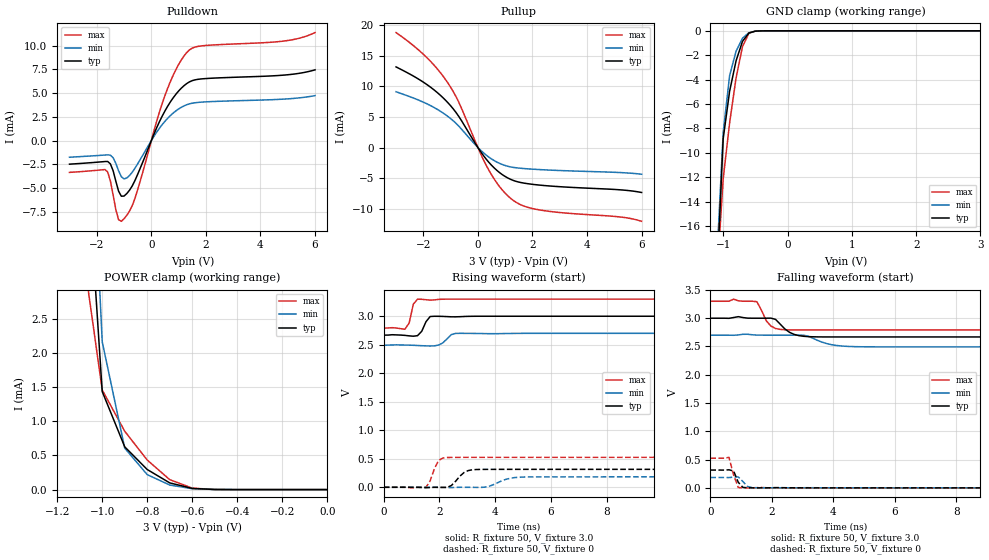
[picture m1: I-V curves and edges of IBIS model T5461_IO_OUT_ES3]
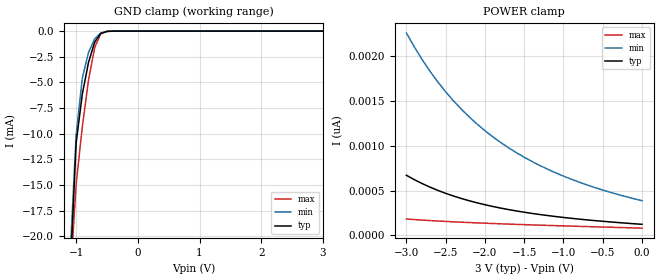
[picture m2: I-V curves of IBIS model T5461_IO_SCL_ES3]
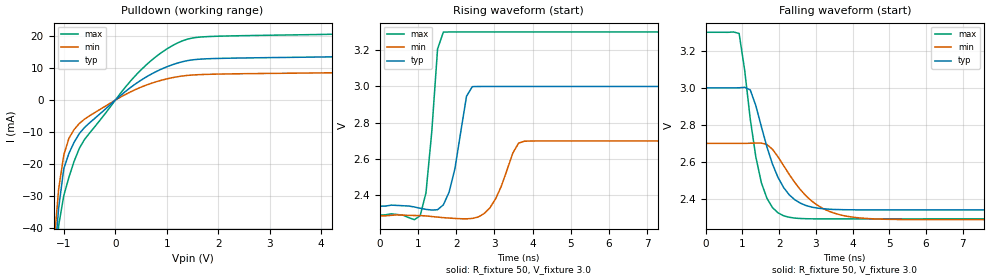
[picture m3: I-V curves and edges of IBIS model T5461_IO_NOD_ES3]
[IBIS Ver]   3.2
[Comment Char]   |_char
[File name]   rx8130ce_3v.ibs
[File Rev]   1.0
[Date]   2019/10/29 15:22:26
[Source]
[Notes]
[Disclaimer]
This information is for modeling purposes only, and is not guaranteed.
Property of SEIKO EPSON Corp.,
unauthorized reproduction and/or distribution is strictly prohibited.
[Copyright]
Copyright 2019, SEIKO EPSON Corp.
[Component]   T5461W0A0
Si_location Pin
Timing_location Pin
[Manufacturer]   SEIKO EPSON Corp.
| RX8130CE
[Package]
R_pkg   0.0m   0.0m   0.0m
L_pkg   0.0n   0.0n   0.0n
C_pkg   0.0p   0.0p   0.0p
[Pin] signal_name   model_name
1   VIO   POWER
2   SCL   T5461_IO_SCL_ES3
3   SDA   T5461_IO_DIO_SMT_ES3
4   FOUT   T5461_IO_OUT_ES3
5   /RST   T5461_IO_NOD_ES3
6   /IRQ   T5461_IO_NOD_ES3
7   GND   POWER
8   VDD   POWER
9   VOUT   POWER
10   VBAT   POWER
| Models and submodels in the file (4): T5461_IO_OUT_ES3 (3-state), T5461_IO_SCL_ES3 (Input), T5461_IO_NOD_ES3 (Open_drain), T5461_IO_DIO_SMT_ES3 (I/O_open_drain)
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[Model]   T5461_IO_OUT_ES3
Model_type 3-state
Enable Active-High
Polarity Non-Inverting
Vmeas=1.50
C_comp   2.5p   2.0p   3.0p
[Temperature Range] 25   85   -40
[Voltage Range]   3.0   2.7   3.3
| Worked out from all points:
|   slope of the pulldown table from 0 to 0.45 V, typ, clamps not added: 157 ohm
|   slope of the pullup table from 0 to 0.45 V, typ, clamps not added: 170 ohm
|   GND clamp passes 1 mA (typ) near -0.71 V on its own axis
|   POWER clamp passes 1 mA (typ) near -0.95 V on its own axis
|   falling waveform, R_fixture 50, V_fixture 3.0: 20-80 % time 437ps typ, 644ps min, 312ps max; typ from 3 V to 2.67 V
|   falling waveform, R_fixture 50, V_fixture 0: 20-80 % time 175ps typ, 196ps min, 177ps max; typ from 0.315 V to 0 V
|   rising waveform, R_fixture 50, V_fixture 3.0: 20-80 % time 204ps typ, 261ps min, 138ps max; typ from 2.67 V to 3 V
|   rising waveform, R_fixture 50, V_fixture 0: 20-80 % time 372ps typ, 557ps min, 264ps max; typ from 0 V to 0.315 V
[Pullup]
-3V       13.15mA    9.1mA      18.76mA
-2V       10.67mA    7.402mA    15.22mA
-1.2V     7.774mA    5.394mA    11.17mA
-700mV    5.069mA    3.488mA    7.383mA
100mV     -670.8uA   -442.9uA   -1.015mA
400mV     -2.405mA   -1.562mA   -3.683mA
800mV     -4.114mA   -2.598mA   -6.416mA
1.3V      -5.375mA   -3.246mA   -8.638mA
1.7V      -5.817mA   -3.436mA   -9.577mA
2.3V      -6.149mA   -3.611mA   -10.21mA
5.2V      -6.899mA   -4.083mA   -11.33mA
6V        -7.339mA   -4.363mA   -12.04mA
[Pulldown]
-3V       -2.479mA   -1.747mA   -3.344mA
-1.6V     -2.194mA   -1.497mA   -3.304mA
-1.4V     -3.175mA   -1.806mA   -5.728mA
-1.2V     -5.321mA   -3.18mA    -8.323mA
-1.1V     -5.852mA   -3.796mA   -8.495mA
-900mV    -5.578mA   -3.932mA   -7.863mA
-600mV    -4.197mA   -2.907mA   -6.073mA
600mV     3.627mA    2.353mA    5.517mA
1.3V      6.014mA    3.781mA    9.282mA
1.8V      6.487mA    4.045mA    9.961mA
4.8V      6.886mA    4.362mA    10.47mA
6V        7.452mA    4.738mA    11.38mA
[GND Clamp]
-3V       -430mA     -359.3mA   -539.8mA
-1.1V     -20.64mA   -18.88mA   -20.39mA
-1V       -8.831mA   -8.329mA   -12.11mA
-900mV    -4.941mA   -3.657mA   -7.543mA
-800mV    -2.459mA   -1.675mA   -3.865mA
-700mV    -864uA     -604.2uA   -1.29mA
-600mV    -179.4uA   -151uA     -195.7uA
-500mV    -26.95uA   -29.51uA   -18.23uA
-400mV    -3.685uA   -4.954uA   -1.653uA
3V        88.91pA    20.06nA    44.45pA
[POWER Clamp]
-3V       324.7mA    274.7mA    407.4mA
-1.1V     6.482mA    9.074mA    3.807mA
-1V       1.434mA    2.163mA    1.457mA
-900mV    625.6uA    606.7uA    853.6uA
-800mV    293.7uA    218.9uA    432uA
-700mV    98.19uA    66.89uA    145.6uA
-600mV    17.36uA    13.33uA    21.68uA
-500mV    1.719uA    1.888uA    1.298uA
0V        88.91pA    301.9pA    52.79pA
[Falling Waveform]
R_fixture=50
V_fixture=3.0
V_fixture_min=2.7
V_fixture_max=3.3
0s        3V         2.7V       3.3V
1.515ns   3V         2.702V     3.292V
1.818ns   3V         2.7V       2.957V
1.97ns    3.001V     2.7V       2.862V
2.121ns   2.979V     2.7V       2.819V
2.424ns   2.811V     2.7V       2.796V
3.03ns    2.681V     2.699V     2.793V
3.939ns   2.669V     2.532V     2.793V
4.697ns   2.668V     2.497V     2.793V
15ns      2.668V     2.493V     2.793V
[Falling Waveform]
R_fixture=50
V_fixture=0
V_fixture_min=0
V_fixture_max=0
0s        314.7mV    183mV      525mV
454.5ps   313.6mV    182.4mV    523.9mV
606.1ps   319.2mV    181.5mV    540.1mV
757.6ps   298.7mV    190.7mV    227.4mV
909.1ps   98.15mV    193.1mV    5.762mV
1.061ns   8.292mV    110.5mV    366.7uV
1.212ns   925.4uV    24.36mV    -21.8uV
1.364ns   103.2uV    4.285mV    329.5uV
1.515ns   -16.13uV   1.324mV    4.103mV
15ns      0V         0V         0V
[Rising Waveform]
R_fixture=50
V_fixture=3.0
V_fixture_min=2.7
V_fixture_max=3.3
0s        2.668V     2.493V     2.793V
757.6ps   2.664V     2.495V     2.772V
909.1ps   2.656V     2.493V     2.877V
1.061ns   2.65V      2.49V      3.212V
1.212ns   2.659V     2.487V     3.299V
1.364ns   2.736V     2.483V     3.297V
1.667ns   2.995V     2.478V     3.283V
1.818ns   2.999V     2.48V      3.287V
2.576ns   2.99V      2.699V     3.3V
15ns      3V         2.7V       3.3V
[Rising Waveform]
R_fixture=50
V_fixture=0
V_fixture_min=0
V_fixture_max=0
0s        0V         0V         0V
1.515ns   -8.195mV   111.8uV    440.3uV
1.667ns   -4.303mV   98.36uV    115mV
1.818ns   -472.6uV   -134.8uV   326.9mV
1.97ns    -1.214mV   -804.1uV   468.6mV
2.273ns   -1.665mV   -4.03mV    521.9mV
2.879ns   257.7mV    -371uV     524.6mV
3.333ns   311.7mV    -2.063mV   524.9mV
5ns       314.7mV    179.3mV    525mV
15ns      314.7mV    183mV      525mV
[Ramp]
R_load=50
dV/dt_r   1.888E-1/3.592E-10   1.098E-1/5.448E-10   3.150E-1/2.380E-10
dV/dt_f   1.989E-1/4.212E-10   1.243E-1/6.375E-10   3.044E-1/2.762E-10
|[End   T5461_IO_OUT_ES3
[Model]   T5461_IO_SCL_ES3
Model_type Input
Enable Active-High
Polarity Non-Inverting
Vinh=2.64
Vinl=0.54
C_comp   2.5p   2.0p   3.0p
[Temperature Range] 25   85   -40
[Voltage Range]   3.0   2.7   3.3
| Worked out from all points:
|   GND clamp passes 1 mA (typ) near -0.69 V on its own axis
[GND Clamp]
-3V       -502.2mA   -418.5mA   -628.9mA
-1.1V     -24.07mA   -22.18mA   -24.54mA
-1V       -10.87mA   -10.09mA   -14.91mA
-900mV    -6.13mA    -4.561mA   -9.309mA
-800mV    -3.058mA   -2.097mA   -4.786mA
-700mV    -1.078mA   -757.4uA   -1.604mA
-600mV    -224.6uA   -189.6uA   -244.1uA
-500mV    -33.81uA   -37.1uA    -22.82uA
-400mV    -4.624uA   -6.222uA   -2.07uA
3V        124.1pA    455.9pA    73.37pA
[POWER Clamp]
-3V       672pA      2.262nA    183.3pA
-2.8V     579.6pA    1.965nA    171.4pA
-2.7V     539.7pA    1.834nA    166pA
-2.5V     470.3pA    1.605nA    156.4pA
-2.4V     440.2pA    1.503nA    152pA
-2.2V     387.4pA    1.324nA    143.9pA
-2V       343.1pA    1.17nA     136.5pA
-1.8V     305.5pA    1.039nA    129.8pA
-1.4V     245.9pA    825.7pA    117.6pA
-1V       200.8pA    662.6pA    106.6pA
-500mV    157.9pA    507.1pA    93.84pA
0V        124.1pA    388pA      81.19pA
[Model]   T5461_IO_NOD_ES3
Model_type Open_drain
Enable Active-High
Polarity Non-Inverting
Vmeas=1.50
Vref=3.3
Rref=5000
C_comp   2.5p   2.0p   3.0p
[Temperature Range] 25   85   -40
[Voltage Range]   3.0   2.7   3.3
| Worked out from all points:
|   slope of the pulldown table from 0 to 0.45 V, typ, clamps not added: 78.7 ohm
|   falling waveform, R_fixture 50, V_fixture 3.0: 20-80 % time 679ps typ, 1.01ns min, 450ps max; typ from 3 V to 2.34 V
|   rising waveform, R_fixture 50, V_fixture 3.0: 20-80 % time 332ps typ, 458ps min, 231ps max; typ from 2.34 V to 3 V
[Pulldown]
-3V       -460.3mA   -383.6mA   -577.8mA
-1.2V     -53.34mA   -46.96mA   -63.7mA
-1.1V     -33.78mA   -27.79mA   -39.25mA
-1V       -21.42mA   -17.13mA   -29.89mA
-900mV    -16.66mA   -11.93mA   -24.12mA
-700mV    -10.51mA   -7.336mA   -15.14mA
-600mV    -8.596mA   -5.984mA   -12.36mA
500mV     6.256mA    4.072mA    9.496mA
900mV     9.765mA    6.259mA    14.95mA
1.3V      12.03mA    7.562mA    18.56mA
1.8V      12.97mA    8.09mA     19.92mA
6V        14.9mA     9.477mA    22.76mA
[Falling Waveform]
R_fixture=50
V_fixture=3.0
V_fixture_min=2.7
V_fixture_max=3.3
0s        3V         2.7V       3.3V
909.1ps   3V         2.7V       3.293V
1.061ns   3.003V     2.7V       3.094V
1.212ns   2.989V     2.701V     2.832V
1.515ns   2.79V      2.701V     2.487V
1.818ns   2.588V     2.668V     2.353V
2.121ns   2.462V     2.58V      2.309V
3.03ns    2.351V     2.368V     2.292V
4.091ns   2.341V     2.3V       2.292V
15ns      2.341V     2.288V     2.292V
[Rising Waveform]
R_fixture=50
V_fixture=3.0
V_fixture_min=2.7
V_fixture_max=3.3
0s        2.341V     2.288V     2.292V
1.061ns   2.329V     2.289V     2.289V
1.212ns   2.324V     2.287V     2.415V
1.515ns   2.322V     2.281V     3.206V
1.667ns   2.348V     2.278V     3.299V
2.273ns   2.946V     2.271V     3.3V
2.424ns   2.999V     2.274V     3.3V
2.879ns   3V         2.33V      3.3V
3.788ns   3V         2.699V     3.3V
15ns      3V         2.7V       3.3V
[Ramp]
R_load=50
dV/dt_r   3.954E-1/3.061E-10   2.472E-1/4.512E-10   6.046E-1/2.163E-10
dV/dt_f   3.954E-1/6.711E-10   2.472E-1/1.010E-9   6.046E-1/4.461E-10
|[End   T5461_IO_NOD_ES3
